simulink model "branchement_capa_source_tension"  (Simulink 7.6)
settings: Solver=ode15s  StartTime=0.0  StopTime=0.015  RelTol=1e-3
StopFcn:
  | close all
  | load VI.mat
  | plotyy(x(1,:),x(2,:),x(1,:),x(3,:))
  | grid
  | title('Tension et courant dans le circuit LC')
  | xlabel('temps')
libraries: powerlib x8

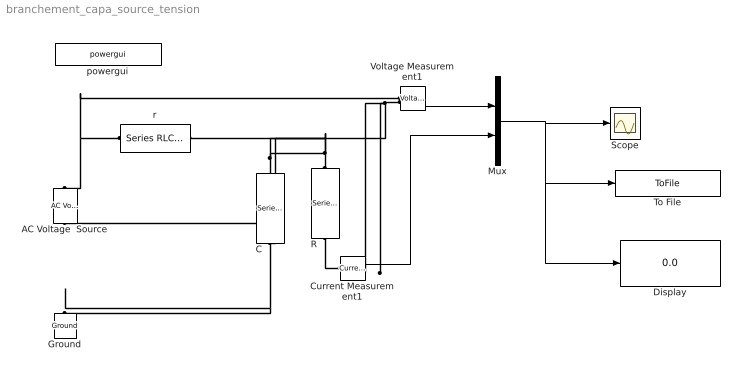
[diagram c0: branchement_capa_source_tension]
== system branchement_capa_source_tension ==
  AC Voltage  Source : powerlib/Electrical Sources/AC Voltage Source  DialogController=POWERSYS.PowerSysDialog  SystemSampleTime=-1  Amplitude=100  Phase=0  Frequency=60  SampleTime=0  Measurements=None
  C : powerlib/Elements/Series RLC Branch  DialogController=POWERSYS.PowerSysDialog  PhysicalDomain=powersysdomain  SubClassName=unknown  LeftPortType=p1  RightPortType=p1  LConnTagsString=__new0  RConnTagsString=__new0  BranchType=C  Resistance=1  Inductance=1e-3  SetiL0=off  InitialCurrent=0  Capacitance=1e-6  Setx0=off  InitialVoltage=0  Measurements=None
  Current Measurement1 : powerlib/Measurements/Current Measurement  DialogController=POWERSYS.PowerSysDialog  SystemSampleTime=-1  PhasorSimulation=off  OutputType=Complex  PSBequivalent=0
  Display : Display
  Ground : powerlib/Elements/Ground  DialogController=POWERSYS.PowerSysDialog  PhysicalDomain=powersysdomain  SubClassName=unknown  LeftPortType=p1  RightPortType=p1  LConnTagsString=a
  Mux : Mux  Inputs=2
  R : powerlib/Elements/Series RLC Branch  DialogController=POWERSYS.PowerSysDialog  PhysicalDomain=powersysdomain  SubClassName=unknown  LeftPortType=p1  RightPortType=p1  LConnTagsString=__new0  RConnTagsString=__new0  BranchType=R  Resistance=10  Inductance=1e-3  SetiL0=off  InitialCurrent=0  Capacitance=1e-6  Setx0=off  InitialVoltage=0  Measurements=None
  Scope : Scope
  To File : ToFile  Filename=VI.mat  MatrixName=x
  Voltage Measurement1 : powerlib/Measurements/Voltage Measurement  DialogController=POWERSYS.PowerSysDialog  SystemSampleTime=-1  PhasorSimulation=off  OutputType=Complex  PSBequivalent=0
  powergui : powerlib/powergui  Priority=1  SystemSampleTime=-1  SimulationMode=Continuous  SampleTime=50e-6  frequency=60  SPID=off  DisableSnubberDevices=off  DisableRonSwitches=off  DisableVfSwitches=off  SwTol=0  Interpol=off  frequencyindice=60  echomessages=off  HookPort=off  DisplayEquations=off  FunctionMessages=off  EnableUseOfTLC=off  x0status=blocks  RestoreLinks=warning  ResistiveCurrentMeasurement=off  Ylog=off  Xlog=on  ShowGrid=off  save=off  variable=ZData  ZoomFFT=off  StartTime=0.0  cycles=1  DisplayStyle=1  fundamental=60  FreqAxis=off  MaxFrequency=1000  frequencyindicesteady=1  display=off  methode=off
  r : powerlib/Elements/Series RLC Branch  DialogController=POWERSYS.PowerSysDialog  PhysicalDomain=powersysdomain  SubClassName=unknown  LeftPortType=p1  RightPortType=p1  LConnTagsString=__new0  RConnTagsString=__new0  BranchType=R  Resistance=100  Inductance=1e-3  SetiL0=off  InitialCurrent=0  Capacitance=1e-6  Setx0=off  InitialVoltage=0  Measurements=None
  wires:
  Voltage Measurement1/1 -> Mux/1
  Mux/1 -> Scope/1, To File/1, Display/1
  Current Measurement1/1 -> Mux/2
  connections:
  R/RConn1 -- C/RConn1 -- r/LConn1
  Voltage Measurement1/LConn2 -- AC Voltage  Source/LConn1 -- Ground/LConn1 -- C/LConn1 -- Current Measurement1/RConn1
  r/RConn1 -- AC Voltage  Source/RConn1 -- Voltage Measurement1/LConn1
  R/LConn1 -- Current Measurement1/LConn1
